{attribute 'qualified_only'}
VAR_GLOBAL
	stPLCtoPMC		:	dut_PLC_to_PMC ;	// PLC传送到PMC数据
	stPMCtoPLC		:	dut_PMC_to_PLC ;	// PMC传送到PLC数据
	
	bAV65Open		:BOOL;
	bAV65Close		:BOOL;
	bAV79Open		:BOOL;
	bAV79Close		:BOOL;
	bAV202Open		: BOOL;
	bAV202Close		: BOOL;
	bAV91Open		:BOOL;
	bAV91Close		:BOOL;
END_VAR
